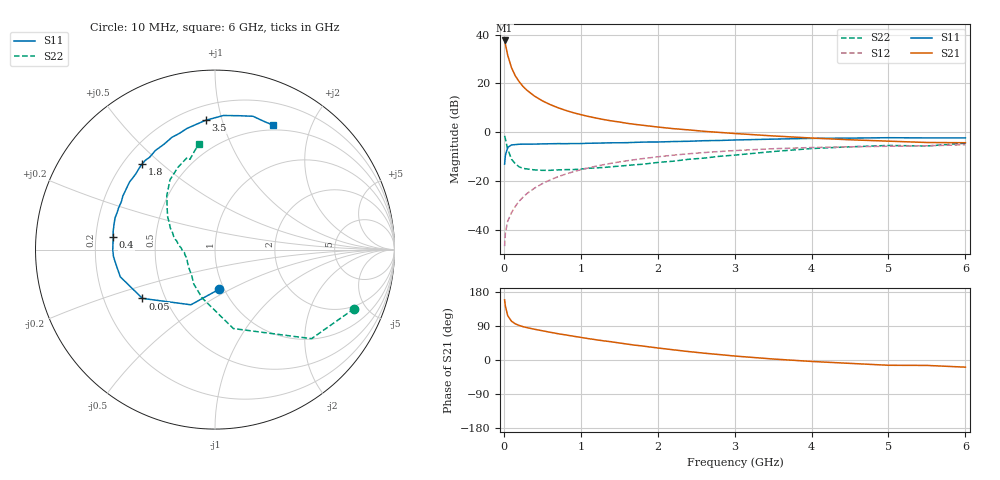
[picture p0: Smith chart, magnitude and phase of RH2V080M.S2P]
! SIEMENS Small Signal Semiconductors
! BFR106
! Si NPN RF Bipolar Junction Transistor in SOT23
! VCE = 2 V  IC = 80 mA
! Common Emitter S-Parameters:  August  1996
# GHz  S  MA  R  50
!  f  S11  S21  S12  S22
! GHz  MAG  ANG  MAG  ANG  MAG  ANG  MAG  ANG
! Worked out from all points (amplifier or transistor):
!   36 points, 10 MHz to 6 GHz, reference 50 ohm
!   highest |S21| = 37.7 dB at 10 MHz (marker M1)
!   |S21| within 3 dB of that: start of sweep to 30.03 MHz
!   unconditionally stable (mu >= 1): 164.7 MHz to 2.933 GHz; 4.922 GHz to end of sweep
!   at 250 MHz: K = 1.06, MAG = 21.2 dB, |S12| = -26.6 dB
!   at 1.4 GHz: K = 1.07, MAG = 7.1 dB, |S12| = -12.7 dB
!   at 6 GHz: K = 1.02, MAG = -0.4 dB, |S12| = -5.1 dB
!   S11 on the Smith chart (normalised r, x): 10 MHz: 0.95, -0.44; 50 MHz: 0.37, -0.27; 400 MHz: 0.27, +0.06; 1.8 GHz: 0.28, +0.43; 3.5 GHz: 0.29, +0.89; 6 GHz: 0.44, +1.48
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0.01  0.2218 -83.9  76.33 158.6  0.0046 77.0  0.8424 -23.0
0.02  0.3355 -113.6  64.5 142.3  0.0086 68.1  0.7318 -42.7
0.05  0.4874 -146.1  38 117.0  0.0149 60.1  0.4517 -76.9
0.1  0.5492 -164.0  20.98 102.2  0.0224 63.2  0.2784 -105.0
0.15  0.5583 -171.8  14.26 95.3  0.0303 68.6  0.2252 -121.8
0.2  0.5671 -176.1  10.85 91.2  0.0386 70.4  0.1947 -131.6
0.25  0.5696 180.0  8.669 87.9  0.0467 71.8  0.1812 -141.1
0.3  0.5693 177.8  7.265 85.5  0.0551 72.7  0.1767 -146.4
0.4  0.5712 173.0  5.493 81.1  0.0716 72.8  0.1686 -155.5
0.5  0.5765 169.7  4.416 77.2  0.0881 72.3  0.1653 -161.5
0.6  0.5801 165.7  3.705 73.3  0.1049 71.5  0.1654 -164.9
0.7  0.5842 162.4  3.201 69.5  0.1215 70.2  0.1686 -168.4
0.9  0.5854 156.4  2.523 62.9  0.1541 67.3  0.1714 -174.8
1.1  0.5942 149.8  2.107 56.4  0.1854 64.1  0.182 -178.5
1.4  0.6074 141.4  1.707 48.0  0.2311 59.0  0.1958 175.1
1.8  0.6266 130.6  1.393 37.0  0.287 52.1  0.2205 166.9
2.2  0.6444 121.0  1.185 27.0  0.3381 45.1  0.2543 158.4
2.8  0.6773 107.0  0.993 14.4  0.4017 34.9  0.3202 145.4
3.5  0.7221 94.2  0.84 2.6  0.4592 23.9  0.4017 132.0
4.5  0.7575 80.0  0.7 -8.9  0.5018 9.7  0.5024 114.3
5.5  0.7643 68.6  0.616 -14.3  0.5267 1.1  0.5221 105.5
6  0.7654 65.0  0.609 -18.9  0.5537 -5.6  0.596 98.8
